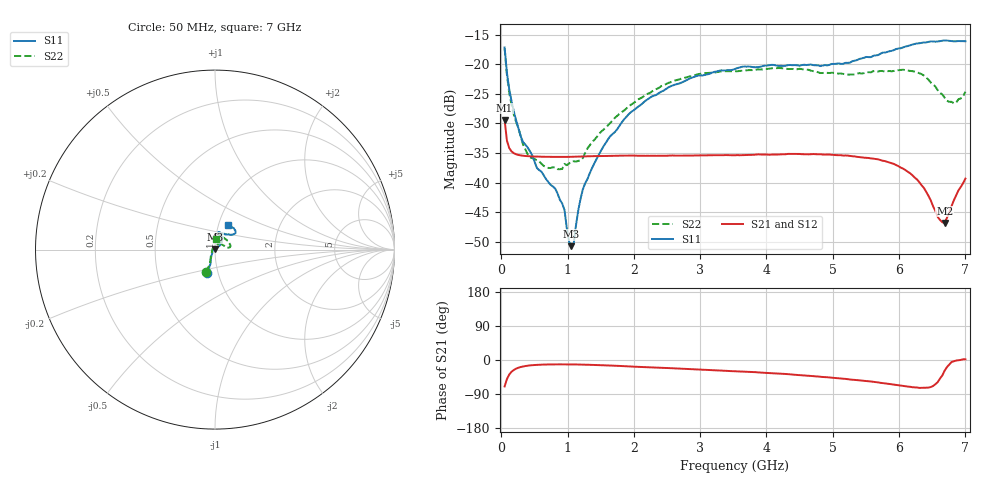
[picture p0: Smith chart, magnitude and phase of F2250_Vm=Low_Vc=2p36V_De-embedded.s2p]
! Integrated Device Technology
! Corporate Headquarters
! 6024 Silver Creek Valley Road
! San Jose, CA 95138  USA
! Phone:  1-408-284-8200
! Toll Free:  1-800-223-1366
! Webpage:  http://www.idt.com/
! Timing and RF Division
! 515 Groton Road, Suite 102
! Westford, MA 01886-6024
! Device:  F2250
! Description: Voltage Variable RF Attenuator
! Frequency:  50.0 -  6000.00 MHz
! Package:  3x3 mm Thin QFN Plastic Package: 16 pin
! Ports:  2 RF, 3 DC
!  Pin  1  = GND
!  Pin  2  = NC
!  Pin  3  = RF1  = Port 1
!  Pin  4  = NC
!  Pin  5  = GND
!  Pin  6  = GND
!  Pin  7  = GND
!  Pin  8  = GND
!  Pin  9  = NC
!  Pin 10  = RF2  = Port 2
!  Pin 11  = NC
!  Pin 12  = GND
!  Pin 13  = GND
!  Pin 14  = VCNTRL
!  Pin 15  = VDD
!  Pin 16  = VMODE
! Vcntrl:  2.360 Volts
! Vmode:  +0.000 Volts
! Vdd:  +3.30  Volts
! Current:  1.176 mA
! Data:  The device was measured on a the F2250 evaluation board which has
!  individual transmission lines to the RF pins.  Data was collected
!  using a calibrated network analyzer.  The evaluation board was
!  de-embedded using a TRL calibration technique.
!  The reference plane is the edge of the package pin.
! Misc:  SN 10
!  Action Tracker AT0258
! Date Measured:  2014-11-26
! Date:  2015-10-15  MJV
! Note:
!  Integrated Device Technology supplies this data as a sample of measured
!  data at the package pin for this product.  Your particular data for this
!  product may vary.
!  Data was taken at 25 degrees C.
!  Integrated Device Technology reserves the right to change this data at anytime.
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# GHz S dB R 50
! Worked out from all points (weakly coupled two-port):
!   201 points, 50 MHz to 7 GHz, reference 50 ohm
!   highest |S21| = -29.41 dB at 50 MHz (marker M1); lowest = -46.8 dB at 6.687 GHz (marker M2)
!   lowest |S11| = -50.8 dB at 1.058 GHz (marker M3), VSWR 1.01, Z = 49.8 + j0.242 ohm
!   |S11| at or under -10 dB: start of sweep to end of sweep
!   |S22| runs from -37.8 to -17.3 dB; largest |S21 - S12| = 5.5e-05
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0.05  -17.18 -108.6  -29.41 -69.8  -29.41 -69.8  -17.29 -110.9
0.08475  -21.45 -107.5  -32.91 -50.3  -32.91 -50.3  -21.77 -110.0
0.15425  -26.23 -116.6  -34.74 -31.1  -34.74 -31.1  -26.86 -122.0
0.29325  -32.21 -127.7  -35.42 -18.4  -35.42 -18.4  -32.19 -136.9
0.3975  -34.09 -141.7  -35.55 -15.0  -35.55 -15.0  -35.21 -160.1
0.91875  -43.55 157.9  -35.67 -11.5  -35.67 -11.5  -37.70 132.6
0.9535  -44.64 170.0  -35.67 -11.5  -35.67 -11.5  -36.84 130.4
1.023  -50.01 144.1  -35.66 -11.6  -35.66 -11.6  -36.78 114.8
1.05775  -50.76 122.9  -35.65 -11.6  -35.65 -11.6  -36.43 109.7
1.0925  -50.32 89.5  -35.64 -11.7  -35.64 -11.7  -36.40 105.2
1.162  -44.64 56.7  -35.63 -11.9  -35.62 -11.8  -36.33 94.3
1.2315  -41.10 44.2  -35.59 -12.1  -35.59 -12.1  -35.84 84.7
1.6485  -32.11 42.0  -35.51 -14.6  -35.51 -14.6  -29.88 63.9
1.9265  -28.40 41.4  -35.46 -16.9  -35.46 -16.9  -27.09 56.3
2.37825  -24.87 47.3  -35.47 -20.3  -35.47 -20.3  -24.00 56.5
3.525  -20.80 72.5  -35.39 -29.6  -35.40 -29.6  -21.22 74.6
4.7065  -20.17 72.4  -35.19 -42.6  -35.19 -42.6  -21.18 72.2
5.85325  -17.82 40.5  -36.63 -63.3  -36.63 -63.3  -21.15 22.8
6.27025  -16.50 40.1  -39.49 -72.6  -39.49 -72.6  -21.37 9.5
6.68725  -15.99 48.8  -46.84 -27.9  -46.81 -27.6  -25.67 28.3
6.861  -16.13 55.1  -42.17 -1.5  -42.13 -1.3  -26.51 57.9
7  -16.12 63.2  -39.34 1.8  -39.31 1.6  -24.65 83.2
